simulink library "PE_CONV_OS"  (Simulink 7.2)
settings: Solver=ode45  SolverMode=SingleTasking  StartTime=0.0  StopTime=10.0  RelTol=1e-3
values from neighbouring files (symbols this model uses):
  C = 10e-3*1    (= 0.01)    [INIT_B6_2L_3Ph_IGBT_OS.m]    (also in INIT_B6_3L_3Ph_IGBT_OS.m; INIT_MMC_100L.m = 0.005; INIT_MMC_200L.m = 0.005; INIT_MMC_20L.m)
  FS = 900    [INIT_B6_2L_3Ph_IGBT_OS.m]    (also in INIT_B6_3L_3Ph_IGBT_OS.m; INIT_PWM_2L.m = 1000; INIT_PWM_3L.m = 1000; INIT_PWM_Con.m = 1000)
  LN = 2e-3    (= 0.002)    [INIT_PWM_2L.m]    (also in INIT_PWM_3L.m; INIT_PWM_Con.m; INIT_MMC_100L.m = 0.025; INIT_MMC_200L.m = 0.025)
  LS = 1e-3    (= 0.001)    [INIT_B6_2L_3Ph_IGBT_OS.m]    (also in INIT_B6_3L_3Ph_IGBT_OS.m; INIT_MMC_100L.m = 0.025; INIT_MMC_200L.m = 0.025; INIT_MMC_20L.m = 0.0025)
  LT = LN    (= 0.025)    [INIT_MMC_100L.m]    (also in INIT_MMC_200L.m; INIT_MMC_20L.m = 0.002; INIT_MMC_400L.m)
  Nc = 100    [INIT_MMC_100L.m]    (also in INIT_MMC_200L.m = 200; INIT_MMC_20L.m = 20; INIT_MMC_400L.m = 400)
  NT = sqrt(3)*340/400    [INIT_MMC_100L.m]    (also in INIT_MMC_200L.m; INIT_MMC_20L.m = sqrt(3); INIT_MMC_400L.m)
  Rg = 1e-3    (= 0.001)    [INIT_MMC_100L.m]    (also in INIT_MMC_200L.m; INIT_MMC_20L.m; INIT_MMC_400L.m)
  RN = 0.1    [INIT_PWM_2L.m]    (also in INIT_PWM_3L.m; INIT_PWM_Con.m; INIT_MMC_100L.m; INIT_MMC_200L.m)
  RT = RN    (= 0.1)    [INIT_MMC_100L.m]    (also in INIT_MMC_200L.m; INIT_MMC_20L.m; INIT_MMC_400L.m)
  UC0 = 600    [INIT_B6_2L_3Ph_IGBT_OS.m]    (also in INIT_B6_3L_3Ph_IGBT_OS.m = 500; INIT_MMC_100L.m = 6800; INIT_MMC_200L.m = 3400; INIT_MMC_20L.m = 5000)
undefined symbols (not defined in the file or in its folder): A, DT, FT, L, O1, O2, PHT, T, Td
libraries: simulink_extras x2
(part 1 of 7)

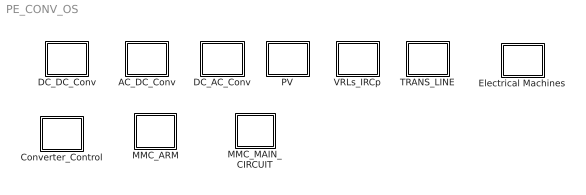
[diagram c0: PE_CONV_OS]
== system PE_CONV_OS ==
  AC_DC_Conv : Subsystem
  Converter_Control : Subsystem
  DC_AC_Conv : Subsystem
  DC_DC_Conv : Subsystem
  Electrical Machines : Subsystem
  MMC_ARM : Subsystem
  MMC_MAIN_CIRCUIT : Subsystem
  PV : Subsystem
  TRANS_LINE : Subsystem
  VRLs_IRCp : Subsystem

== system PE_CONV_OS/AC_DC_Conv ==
  B12D_OS : Subsystem  mask{LS=1e-4, nyy=1, nyd=sqrt(3), LT=1e-4, LD=1e-3, ILD0=200, C=1e-3, VC0=600, RL=2}
      mask prompts: LS "Source Inductance"; nyy "Trafo YY turns Ratio"; nyd "Trafo YD turns Ratio"; LT "Transformer Inductance"; LD "DC Inductance"; ILD0 "Initial Current ILD0"; C "Load Capacitance"; VC0 "Initial Cap Voltage"; RL "Load Resistance"
      mask help: 12-Pulse Diode Bridge Converter Input Vector u: u[0]= Vs1.v u[1]= Vs2.v u[2]= Vs3.v u[3]= IDC1.i u[4]= IDC2.i Output Vector y: y[0]= D11.I y[1]= D11.V y[2]= D12.I y[3]= D12.V y[4]= Lc1.I y[5]= Lc2.I y[6]= Lc3.I y[7]= Ld1.I y[8]= Ld2.I y[9]= VDC1.V y[10]= VDC2.V y[11]= VC1.V y[12]= VC2.V Parameter Vector p: p[0]= Lc1.L p[0]= Lc2.L p[0]= Lc3.L p[1]= nyy p[2]= nyd p[3]= LT.L p[4]= Ld.L p[5]= Ld.IL0 p[6]= C1.C p[7]= C1.vC0 p[8]= R1.r You can pause the simulation during running, change the Parameters you want and continue the Simulation
  B12T_OS : Subsystem  mask{LS=1e-4, LT1=1e-4, LT2=1e-4, LD=1e-3, ILD0=200, C=5e-3, VC0=500, RL=2}
      mask prompts: LS "source Inductance"; LT1 "TYY leakage Inductance"; LT2 "TYD leakage Inductance"; LD "DC Inductance"; ILD0 "Initial Current ILD0"; C "Load Capacitance"; VC0 "Initial Cap Voltage"; RL "Load Resistance"
      mask help: 12-Pulse Thyristor Bridge Converter Input Vector u: u[0]= B6T1_H1.gate u[1]= B6T1_H2.gate u[2]= B6T1_H3.gate u[3]= B6T1_H4.gate u[4]= B6T1_H5.gate u[5]= B6T1_H6.gate u[6]= B6T2_H1.gate u[7]= B6T2_H2.gate u[8]= B6T2_H3.gate u[9]= B6T2_H4.gate u[10]= B6T2_H5.gate u[11]= B6T2_H6.gate u[12]= Vs1.v u[13]= Vs2.v u[14]= Vs3.v u[15]= IDC1.i u[16]= IDC1.i Output Vector y: y[0]= B6T1_T11.I y[1]= B6T1_T11.V y[2]= B6T2_T11.I y[3]= B6T2_T11.V y[4]= Ls1.I y[5]= Ls2.I y[6]= Ls3.I y[7]= Ld1.I y[8]= Ld2.I y[6]= VDC.V y[9]= VC1.V y[10]= VC2.V Parameter Vector p: p[0]= Ls.L p[1]= TYY_LT.L p[2]= TYD_LT.L p[3]= Ld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
  B2D_OS : Subsystem  mask{LS=1e-3, LD=1e-3, ILD0=80, C=1e-5, VC0=80, RD=2}
      mask prompts: LS "Source Inductance"; LD "Load Inductance"; ILD0 "initial  Load Inductance Current"; C "Load Cap"; VC0 "initial Cap Voltage"; RD "Load Resistance"
      mask help: Open Source 2-Pulse Diode Bridge Converter Input Vector u: u[0]= Vs.v u[1]= IDC.i Output Vector y: y[0]= D1.I y[1]= D1.V y[2]= Lc.I y[3]= Ld.I y[4]= VDC.V y[5]= VC.V Parameter Vector p: p[0]= Lc.L p[1]= Ld.L p[2]= Ld.IL0 p[3]= C1.C p[4]= C1.vC0 p[5]= R1.r You can pause the simulation during running, change the Parameters you want and continue the Simulation
  B2T_OS : Subsystem  mask{LS=1e-4, LD=10e-3, ILD0=0, C=10e-3, VC0=100, RL=1}
      mask prompts: LS "Source Inductance"; LD "DC Inductance"; ILD0 "Initial current ILD0"; C "Load Cap"; VC0 "Initial Cap Voltage"; RL "Load Resistance"
      mask help: 2-Pulse Thyristor Bridge Converter Input Vector u: u[0]= H1.gate,H4.gate u[1]= H2.gate,H3.gate u[2]= Vs.v u[3]= IDC.i Output Vector y: y[0]= T1.I y[1]= T1.V y[2]= Lc.I y[3]= Ld.I y[4]= VDC.V y[5]= VC.V Parameter Vector p: p[0]= Lc.L p[1]= Ld.L p[2]= Ld.IL0 p[3]= C1.C p[4]= C1.vC0 p[5]= R1.r You can pause the simulation during running, change the Parameters you want and continue the Simulation
  B2_2L_IGBT_OS : Subsystem  mask(B2-2-Level IGBT Converter){LS=2e-3, C=10e-3, VC0=400, RL=10e5}
      mask prompts: LS "Source Inductance"; C "Load Cap"; VC0 "Initial Cap Voltage"; RL "Load Resistance"
      mask help: Input Vector u: u[0]= IGBT1.gate u[1]= IGBT2.gate u[2]= IGBT3.gate u[3]= IGBT4.gate u[4]= V1.V u[5]= IDC.i Output Vector y: y[0]= T1.I y[1]= D1.I y[2]= T1.V y[3]= T2.I y[4]= D2.I y[5]= T2.V y[6]= LS1.I y[7]= DC.V y[8]= Va.V Parameter Vector p: p[0]= Ls.L p[1]= C1.C p[2]= C1.vC0 p[3]= R1.r You can pause the simulation during running, change the Parameters you want and continue the Simulation
  B2_3LD_IGBT_OS : Subsystem  mask(B2-2-Level IGBT Converter){LS=2e-3, C=10e-3, VC0=200, RL=10e5}
      mask prompts: LS "Source Inductance"; C "Load Cap"; VC0 "Initial Cap Voltage"; RL "Load Resistance"
      mask help: Input Vector u: u[0]= IGBT1.gate u[1]= IGBT2.gate u[2]= IGBT3.gate u[3]= IGBT4.gate u[4]= V1.V u[5]= IDC.i Output Vector y: y[0]= T1.I y[1]= D1.I y[2]= T1.V y[3]= T2.I y[4]= D2.I y[5]= T2.V y[6]= LS1.I y[7]= DC.V y[8]= Va.V Parameter Vector p: p[0]= Ls.L p[1]= C1.C p[2]= C1.vC0 p[3]= R1.r You can pause the simulation during running, change the Parameters you want and continue the Simulation
  B2_3LT_IGBT_OS : Subsystem  mask(B2-2-Level IGBT Converter){LS=2e-3, C=10e-3, VC0=200, RL=10e5}
      mask prompts: LS "Source Inductance"; C "Load Cap"; VC0 "Initial Cap Voltage"; RL "Load Resistance"
      mask help: Input Vector u: u[0]= IGBT1.gate u[1]= IGBT2.gate u[2]= IGBT3.gate u[3]= IGBT4.gate u[4]= V1.V u[5]= IDC.i Output Vector y: y[0]= T1.I y[1]= D1.I y[2]= T1.V y[3]= T2.I y[4]= D2.I y[5]= T2.V y[6]= LS1.I y[7]= DC.V y[8]= Va.V Parameter Vector p: p[0]= Ls.L p[1]= C1.C p[2]= C1.vC0 p[3]= R1.r You can pause the simulation during running, change the Parameters you want and continue the Simulation
  B6D_OS : Subsystem  mask{LS=1e-4, LD=1e-3, ILD0=200, C=1e-3, VC0=500, RL=2}
      mask prompts: LS "Source Inductance"; LD "DC Inductance"; ILD0 "Initial current ILD0"; C "Load Cap"; VC0 "Initial Cap Voltage"; RL "Load Resistance"
      mask help: 6-Pulse Diode Bridge Converter Input Vector u: u[0]= Vs1.v u[1]= Vs2.v u[2]= Vs3.v u[3]= IDC.i Output Vector y: y[0]= D1.I y[1]= D1.V y[2]= Lc1.I y[3]= Lc2.I y[4]= Lc3.I y[5]= Ld.I y[6]= VDC.V y[7]= VC.V Parameter Vector p: p[0]= Lc1.L p[0]= Lc2.L p[0]= Lc3.L p[1]= Ld.L p[2]= Ld.IL0 p[3]= C1.C p[4]= C1.vC0 p[5]= R1.r You can pause the simulation during running, change the Parameters you want and continue the Simulation
  B6T_OS : Subsystem  mask{LS=1e-4, LD=1e-3, ILD0=200, C=2e-3, VC0=500, RL=2}
      mask prompts: LS "Source Inductance"; LD "DC Inductance LD"; ILD0 "Initial current ILD0"; C "Load Cap"; VC0 "Initial Cap Voltage"; RL "Load Resistance"
      mask help: 6-Pulse Thyristor Bridge Converter Input Vector u: u[0]= H1.gate u[1]= H2.gate u[2]= H3.gate u[3]= H4.gate u[4]= H5.gate u[5]= H6.gate u[6]= Vs1.v u[7]= Vs2.v u[8]= Vs3.v u[9]= IDC.i Output Vector y: y[0]= T11.I y[1]= T11.V y[2]= Lc1.I y[3]= Lc2.I y[4]= Lc3.I y[5]= Ld.I y[6]= VDC.V y[7]= VC.V Parameter Vector p: p[0]= Lc.L p[1]= Ld.L p[2]= Ld.IL0 p[3]= C1.C p[4]= C1.vC0 p[5]= R1.r You can pause the simulation during running, change the Parameters you want and continue the Simulation
  B6_2L_3ph_IS_IGBT_OS : Subsystem  mask(B6 2-Level IGBT 3-Phase Converter){C=C, UC0=UC0, RL=10000}
      mask prompts: C "Load Cap"; UC0 "Initial Cap Voltage"; RL "Load Resistance"
      mask help: Input Vector u: u[0]= IGBT1.gate u[1]= IGBT2.gate u[2]= IGBT3.gate u[3]= IGBT4.gate u[4]= IGBT5.gate u[5]= IGBT6.gate u[6]= I1.V u[7]= I2.V u[8]= I3.V u[9]= IDC Output Vector y: y[0]= T1.I y[1]= D1.I y[2]= T1.V y[3]= T2.I y[4]= D2.I y[5]= T2.V y[6]= DC.V y[7]= Va.V y[9]= Vb.V y[10]= Vc.V Parameter Vector p: p[0]= C1.C p[1]= C1.vC0 p[2]= R1.r You can pause the simulation during running, change the Parameters you want and continue the Simulation
  B6_2L_3ph_VLS_IGBT_OS : Subsystem  mask(B6 2-Level IGBT 3-Phase Converter){LS=LS, C=C, UC0=UC0, RL=10000}
      mask prompts: LS "Source Inductance"; C "Load Cap"; UC0 "Initial Cap Voltage"; RL "Load Resistance"
      mask help: Input Vector u: u[0]= IGBT1.gate u[1]= IGBT2.gate u[2]= IGBT3.gate u[3]= IGBT4.gate u[4]= IGBT5.gate u[5]= IGBT6.gate u[6]= V1.V u[7]= V2.V u[8]= V3.V u[9]= IDC.i Output Vector y: y[0]= T1.I y[1]= D1.I y[2]= T1.V y[3]= T2.I y[4]= D2.I y[5]= T2.V y[6]= LS1.I y[7]= LS2.I y[8]= LS3.I y[9]= DC.V y[10]= Va.V y[11]= Vb.V y[12]= Vc.V Parameter Vector p: p[0]= Ls.L p[1]= C1.C p[2]= C1.vC0 p[3]= R1.r You can pause the simulation during running, change the Parameters you want and continue the Simulation
  B6_3LD_3-ph_IGBT_OS : Subsystem  mask(6-Pulse 3-LD IGBT 3-Phase Converter){LS=LS, C=C, VC0=UC0, RL=1000}
      mask prompts: LS "Source Inductance"; C "Load Cap"; VC0 "Initial Cap Voltage"; RL "Load Resistance"
      mask help: Input Vector u: u[0]= IGBT1.gate u[1]= IGBT2.gate u[2]= IGBT3.gate u[3]= IGBT4.gate u[4]= IGBT5.gate u[5]= IGBT6.gate u[6]= IGBT7.gate u[7]= IGBT8.gate u[8]= IGBT9.gate u[9]= IGBT10.gate u[10]= IGBT11.gate u[11]= IGBT12.gate u[12]= V1.V u[13]= V2.V u[14]= V3.V u[15]= IDC.i Output Vector y: y[0]= T1.I y[1]= D1.I y[2]= T1.V y[3]= T2.I y[4]= D2.I y[5]= T2.V y[6]= LS1.I y[7]= LS2.I y[8]= LS3.I y[9]= DC1.V y[10]= DC2.V y[11]= Vab.V Parameter Vector p: p[0]= Ls.L p[1]= C1.C p[2]= C1.vC0 p[3]= R1.r You can pause the simulation during running, change the Parameters you want and continue the Simulation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
  B6_3LT_3-ph_IGBT_OS : Subsystem  mask(6-Pulse 3-LT IGBT 3-Phase Converter){LS=LS, C=C, VC0=UC0, RL=1000}
      mask prompts: LS "Source Inductance"; C "Load Cap"; VC0 "Initial Cap Voltage"; RL "Load Resistance"
      mask help: Input Vector u: u[0]= IGBT1.gate u[1]= IGBT2.gate u[2]= IGBT3.gate u[3]= IGBT4.gate u[4]= IGBT5.gate u[5]= IGBT6.gate u[6]= IGBT7.gate u[7]= IGBT8.gate u[8]= IGBT9.gate u[9]= IGBT10.gate u[10]= IGBT11.gate u[11]= IGBT12.gate u[12]= V1.V u[13]= V2.V u[14]= V3.V u[15]= IDC.i Output Vector y: y[0]= T1.I y[1]= D1.I y[2]= T1.V y[3]= T2.I y[4]= D2.I y[5]= T2.V y[6]= LS1.I y[7]= LS2.I y[8]= LS3.I y[9]= DC1.V y[10]= DC2.V y[11]= Vab.V Parameter Vector p: p[0]= Ls.L p[1]= C1.C p[2]= C1.vC0 p[3]= R1.r You can pause the simulation during running, change the Parameters you want and continue the Simulation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

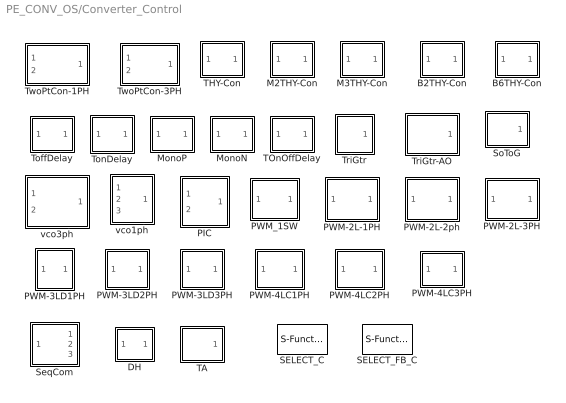
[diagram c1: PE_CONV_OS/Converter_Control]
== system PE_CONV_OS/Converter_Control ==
  B2THY-Con : Subsystem  mask(B2THY-Con){F=50, PH=90, TD=1e-3}
      mask prompts: F "Frequency"; PH "Phase Angle (Degree)"; TD "Puls Duration"
      mask help: Control of one Thyristor in a line commutated Converter circuit
      mask init:
      | x=0:pi/20:2*pi;
      | y=cos(x);
  B6THY-Con : Subsystem  mask(B6THY-Con){F=50, PH=60, TD=1e-3}
      mask prompts: F "Frequency"; PH "Phase Angle (Degree)"; TD "Puls Duration"
      mask help: Control of one Thyristor in a line commutated Converter circuit
      mask init:
      | x=0:pi/20:2*pi;
      | y=cos(x);
  DH : Subsystem
  M2THY-Con : Subsystem  mask(M1THY-Con){F=50, PH=90, TD=1e-3}
      mask prompts: F "Frequency"; PH "Phase Angle (Degree)"; TD "Puls Duration"
      mask help: Control of one Thyristor in a line commutated Converter circuit
      mask init:
      | x=0:pi/20:2*pi;
      | y=cos(x);
  M3THY-Con : Subsystem  mask(M3THY-Con){F=50, PH=60, TD=1e-3}
      mask prompts: F "Frequency"; PH "Phase Angle (Degree)"; TD "Puls Duration"
      mask help: Control of one Thyristor in a line commutated Converter circuit
      mask init:
      | x=0:pi/20:2*pi;
      | y=cos(x);
  MonoN : Subsystem  mask(MonoN){PW=1e-6}
      mask prompts: PW "Pulse Width"
      mask help: Mono Flip Flop on nagative going signal
  MonoP : Subsystem  mask(MonoP){PW=1e-6}
      mask prompts: PW "Pulse Width"
      mask help: Mono Flip Flop on positive going signal
  PIC : Subsystem  mask(PI-controller){Kp=1, Ki=10, lim=15, Ts=-1}
      mask prompts: Kp "Proportional gain (Kp)"; Ki "Integral gain (Ki)"; lim "Output limit"; Ts "Sampling time (s)"
      mask help: Proportional-Integral Controller
  PWM-2L-1PH : Subsystem  mask(PWM-2L-1PH){FT=5000, PHT=0, DT=1e-6}
      mask prompts: FT "Triangular Frequency"; PHT "Trian. Phase Angle (Degree)"; DT "Dead Time"
      mask help: Pulse Width Modulation for 1 Leg of 2-Level Converter
  PWM-2L-2ph : Subsystem  mask(PWM-2L-2PH){FT=500, PHT=0, DT=1e-6}
      mask prompts: FT "Triangular Frequency"; PHT "Trian. Phase Angle (Degree)"; DT "Dead Time"
      mask help: Pulse Width Modulation for 2 Legs of 2-Level Converter
  PWM-2L-3PH : Subsystem  mask(PWM3-2L-3PH){FT=500, PHT=0, DT=1e-6}
      mask prompts: FT "Triangular Frequency"; PHT "Trian. Phase Angle (Degree)"; DT "Dead Time"
      mask help: Pulse Width Modulation for 3 Phase Converter
  PWM-3LD1PH : Subsystem  mask(PWM-3LD_1PH){FT=FT, PHT=PHT, A=A, O1=O1, O2=O2, DT=DT}
      mask prompts: FT "Frequency of Trian Sig."; PHT "Phase Angle of Trian. Sig."; A "Amplitude of Trian. Sig."; O1 "Offset of 1st Trian"; O2 "Offset of 2nd Trian."; DT "Dead Time"
      mask help: Pulse Width Modulation for 1 Leg of 3 Level Neutral point clamped Converter
  PWM-3LD2PH : Subsystem  mask(PWM-3LD_3PH){FT=5000, PHT=0, A=0.5, O1=0.5, O2=-0.5, DT=1e-6}
      mask prompts: FT "Frequency of Trian Sig."; PHT "Phase Angle of Trian. Sig."; A "Amplitude of Trian. Sig."; O1 "Offset of 1st Trian"; O2 "Offset of 2nd Trian."; DT "Dead Time"
      mask help: Pulse Width Modulation for 2 Legs of 3 Level Neutral point clamped Converter
  PWM-3LD3PH : Subsystem  mask(PWM-3LD3PH){FT=500, PHT=0, A=0.5, O1=0.5, O2=-0.5, DT=1e-6}
      mask prompts: FT "Frequency of Trian Sig."; PHT "Phase Angle of Trian. Sig."; A "Amplitude of Trian. Sig."; O1 "Offset of 1st Trian"; O2 "Offset of 2nd Trian."; DT "Dead Time"
      mask help: Pulse Width Modulation for 3 Phase 3 Level Neutral point clamped Converter
  PWM-4LC1PH : Subsystem  mask(PWM-4LC1PH){FT=500, PHT1=0, PHT2=-120, PHT3=-240, DT=1e-6}
      mask prompts: FT "Frequency of Trian Sig."; PHT1 "Phase Angle of 1st Trian. Sig."; PHT2 "Phase Angle of 2nd Trian. Sig."; PHT3 "Phase Angle of 3rd Trian. Sig."; DT "Dead Time"
      mask help: Pulse Width Modulation for 1 Phase 4 Level Floating Capacitor Converter
  PWM-4LC2PH : Subsystem  mask(PWM-4LC1PH){FT=500, PHT1=0, PHT2=-120, PHT3=-240, DT=1e-6}
      mask prompts: FT "Frequency of Trian Sig."; PHT1 "Phase Angle of 1st Trian. Sig."; PHT2 "Phase Angle of 2nd Trian. Sig."; PHT3 "Phase Angle of 3rd Trian. Sig."; DT "Dead Time"
      mask help: Pulse Width Modulation for 1 Phase 4 Level Floating Capacitor Converter
  PWM-4LC3PH : Subsystem  mask(PWM-4LC3PH){FT=500, PHT1=0, PHT2=-120, PHT3=-240, DT=1e-6}
      mask prompts: FT "Frequency of Trian Sig."; PHT1 "Phase Angle of 1st Trian. Sig."; PHT2 "Phase Angle of 2nd Trian. Sig."; PHT3 "Phase Angle of 3rd Trian. Sig."; DT "Dead Time"
      mask help: Pulse Width Modulation for 3 Phases 4 Level Floating Capacitor Converter
  PWM_1SW : Subsystem  mask(PWMtr){FS=1000}
      mask prompts: FS "Frequency"
      mask help: PWM based on Saw tooth Generator
  SELECT_C : S-Function  FunctionName=SELECT_MMC_C  Parameters=2*Nc  EnableBusSupport=off
  SELECT_FB_C : S-Function  FunctionName=SELECT_MMC_AFB_C  Parameters=2*Nc  EnableBusSupport=off
  SeqCom : Subsystem  mask{T=0.02, BF=1024*10}
      mask prompts: T "Period Time"; BF "Beffer Size"
      mask help: Unbalaced 3-phase system to Positive, Negative and Zero Sequence Systems
  SoToG : Subsystem  mask(SoToG){T=1e-3}
      mask prompts: T "Period Time"
      mask help: Saw tooth Generator Input: Period Time
  TA : Subsystem  mask(TriGtr-AO){A=0.5, O=0.5, T=1/FS, Nc=Nc}
      mask prompts: A "Amplitude"; O "Offset"; T "Period Time"; Nc "Output width"
      mask help: Triangular Wave Generator with variable No. of triagles, variable amplitude and offset
  THY-Con : Subsystem  mask(THY-Con){F=50, PH=90, TD=1e-3}
      mask prompts: F "Frequency"; PH "Phase Angle (Degree)"; TD "Puls Duration"
      mask init:
      | x=0:pi/20:2*pi;
      | y=cos(x);
  TOnOffDelay : Subsystem  mask(TOnOffDelay){DT_OFF=1e-6, DT_ON=1e-6}
      mask prompts: DT_OFF "TOffDelay"; DT_ON "TOnDelay"
  ToffDelay : Subsystem  mask(TOffDelay){DT=1e-6}
      mask prompts: DT "TOffDelay"
  TonDelay : Subsystem  mask(TonDelay){DT=1e-6}
      mask prompts: DT "Dead Time"
      mask help: Turn on dead time to protect against short circuit of the converter leg
  TriGtr : Subsystem  mask(TriGtr){T=1e-3, Td=0.0002}
      mask prompts: T "Period Time"; Td "Time Delay"
      mask help: Triangular Wave Generator with variable time delay
  TriGtr-AO : Subsystem  mask(TriGtr-AO){A=0.5, O=0.5, T=T, Td=Td}
      mask prompts: A "Amplitude"; O "Offset"; T "Period Time"; Td "Time Delay"
      mask help: Triangular Wave Generator with variable time delay, variable amplitude and offset
  TwoPtCon-1PH : Subsystem  mask(TwoPtCon-1PH){SP=5, SN=-5, DT=1e-6}
      mask prompts: SP "Positive Limit"; SN "Negative Limit"; DT "Dead Time"
      mask help: Two Point Controller with Dead Time protection for 1Phase Converter
  TwoPtCon-3PH : Subsystem  mask(TwoPtCon-3PH){SP=5, SN=-5, DT=1e-6}
      mask prompts: SP "Positive Limit"; SN "Negative Limit"; DT "Dead Time"
      mask help: Two Point Controller with Dead Time protection for 3 Phase Converter
  vco1ph : Subsystem
  vco3ph : Subsystem

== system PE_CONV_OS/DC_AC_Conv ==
  PWM_2L_3PH_IS : Subsystem
  PWM_2L_3PH_VLR : Subsystem  mask(pwm_2L_3PH_VLR_OS){RL=0.5, LL=1e-3}
      mask prompts: RL "Load R"; LL "Load L"
      mask help: Open Source 2-Level PWM_3PH Converter with VLR load Input Vector u: u[0]= TD1.gate u[1]= TD2.gate u[2]= TD3.gate u[3]= TD4.gate u[4]= TD5.gate u[5]= TD6.gate u[6]= VDC u[7]= Ea, Phase A Load Voltage u[8]= Eb, Phase B Load Voltage u[9]= Ec, Phase C Load Voltage Output Vector y: y[0]= Va.v, Phase A Output Voltage to middle point y[1]= Vb.V, Phase B Output Voltage to middle point y[2]= Vc.V, Phase C Output Voltage to middle point y[3]= Ia.I, Phase A Output AC Current y[4]= Ib.I, Phase B Output AC Current y[5]= Ic.I, Phase C Output AC Current y[6]= Vab.V, Output AC line Voltage y[7]= T1.I y[8]= D1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
  PWM_2L_FB_IS : Subsystem
  PWM_2L_FB_VLR : Subsystem  mask(pwm_2L_FB_VLR_OS){RL=1, LL=1e-3}
      mask prompts: RL "Load R"; LL "Load L"
      mask help: Open Source 2-Level FB_PWM Converter with VLR load Input Vector u: u[0]= TD1.gate u[1]= TD2.gate u[2]= TD3.gate u[3]= TD4.gate u[4]= VDC u[5]= EL, Load Voltage Output Vector y: y[0]= Va.v, Output Voltage to middle point y[1]= Ia.I, Output AC Current y[2]= Vab.V, Output AC Voltage y[3]= T1.I y[4]= D1.I y[5]= T1.V y[6]= DC.I, Input DC Current Parameter Vector p: p[0]= RL p[1]= LL You can pause the simulation during running, change the Parameters you want and continue the Simulation
  PWM_2L_HB_IS : Subsystem
  PWM_2L_HB_VLR : Subsystem  mask(pwm_2L_HB_VLR_OS){RL=0.5, LL=1e-3}
      mask prompts: RL "Load R"; LL "Load L"
      mask help: Open Source 2-Level HB_PWM Converter with VLR load Input Vector u: u[0]= TD1.gate u[1]= TD2.gate u[2]= VDC u[3]= Ea Output Vector y: y[0]= Va.v, Output Voltage to middle point y[1]= Ia.I, Output AC Current y[2]= T1.I y[3]= D1.I y[4]= T1.V y[5]= DC.I, Input DC Current Parameter Vector p: p[0]=RL p[1]=LL You can pause the simulation during running, change the Parameters you want and continue the Simulation
  PWM_3LD_3PH_IS : Subsystem
  PWM_3LD_3PH_VLR : Subsystem  mask(pwm_3LD_3PH_VLR_OS){RL=1, LL=1e-3}
      mask prompts: RL "Load Resistance"; LL "Load Inductance"
      mask help: Open Source 3-Level NPC PWM_3PH Converter with VLR load Input Vector u: u{0:11}= gating Signals u[12]/2= VDC1, VDC2 u{13:15}= EA,EB,EC Output Vector y: y{0:2}= Va,Vb,Vc, Output AC Voltages to middle point y{3:5}= Ia,Ib,Ic, Output AC Currents y[6]= Vab.V, Output Voltage y{7:9} = T1.I,D1.I,T1.V y{10:12}= T2.I,D2.I,T2.V y[13]= D5.I y[14]= D5.V y[15]= IDC1, Input DC Current y[16]= IDC2, Input DC Current Parameter Vector p: p[0]=RL p[1]=LL You can pause the simulation during running, change the Parameters you want and continue the Simulation
  PWM_3LD_FB_IS : Subsystem
  PWM_3LD_FB_VLR : Subsystem  mask(pwm_3LD_FB_VLR_OS){RL=1, LL=1e-3}
      mask prompts: RL "Load Resistance"; LL "Load Inductance"
      mask help: Open Source 3-Level NPC Full Bridge Converter with VLR load Input Vector u: u[0]= L3L1_TD1.gate u[1]= L3L1_TD2.gate u[2]= L3L1_TD3.gate u[3]= L3L1_TD4.gate u[4]= L3L2_TD1.gate u[5]= L3L2_TD2.gate u[6]= L3L2_TD3.gate u[7]= L3L2_TD4.gate u[8]= VDC u[9]= EL Output Vector y: y[0]= Va.v, Output AC Voltage to middle point y[1]= Ia.I, Output AC Current y[2]= Vab.V, Output AC Voltage y[3]= T1.I y[4]= D1.I y[5]= T1.V y[6]= T2.I y[7]= D2.I y[8]= T2.V y[9]= D5.I y[10]= D5.V y[11]= IDC1, Input DC Current y[12]= IDC2, Input DC Current Parameter Vector p: p[0]=RL p[1]=LL You can pause the simulation during 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
  PWM_3LD_HB_IS : Subsystem
  PWM_3LD_HB_VLR : Subsystem  mask(pwm_3LD_HB_VLR_OS){RL=0.5, LL=2e-3}
      mask prompts: RL "Load Resistance"; LL "Load Inductance"
      mask help: Open Source 3-Level NPC PWM HB Converter with VLR load Input Vector u: u[0]= L3L1_TD1.gate u[1]= L3L1_TD2.gate u[2]= L3L1_TD3.gate u[3]= L3L1_TD4.gate u[4]= VDC u[5]= Ea Output Vector y: y[0]= Va.v, Output Voltage to middle point y[1]= Ia.I, Output AC Current y[2]= T1.I y[3]= D1.I y[4]= T1.V y[5]= T2.I y[6]= D2.I y[7]= T2.V y[8]= D5.I y[9]= D5.V y[10]= IDC1, Input DC Current y[11]= IDC2, Input DC Current Parameter Vector p: p[0]=RL p[1]=LL You can pause the simulation during running, change the Parameters you want and continue the Simulation
  PWM_3LT_3PH_IS : Subsystem
  PWM_3LT_3PH_VLR : Subsystem  mask(pwm_3LT_3PH_VLR_OS){RL=1, LL=1e-3}
      mask prompts: RL "Load Resistance"; LL "Load Inductance"
      mask help: Open Source 3-Level T-NPC PWM_3PH Converter with VLR load Input Vector u: u{0:11}= gating Signals u[12]/2= VDC1, VDC2 u{13:15}= EA,EB,EC Output Vector y: y{0:2}= Va,Vb,Vc, Output AC Voltages to middle point y{3:5}= Ia,Ib,Ic, Output AC Currents y[6]= Vab.V, Output Voltage y{7:9} = T1.I,D1.I,T1.V y{10:12}= T2.I,D2.I,T2.V y[13]= D5.I y[14]= D5.V y[15]= IDC1, Input DC Current y[16]= IDC2, Input DC Current Parameter Vector p: p[0]=RL p[1]=LL You can pause the simulation during running, change the Parameters you want and continue the Simulation
  PWM_3LT_FB_IS : Subsystem
  PWM_3LT_FB_VLR : Subsystem  mask(pwm_3LT_FB_VLR_OS){RL=1, LL=1e-3}
      mask prompts: RL "Load Resistance"; LL "Load Inductance"
      mask help: Open Source 3-Level T-NPC Full Bridge Converter Input Vector u: u[0]= L3L1_TD1.gate u[1]= L3L1_TD2.gate u[2]= L3L1_TD3.gate u[3]= L3L1_TD4.gate u[4]= L3L2_TD1.gate u[5]= L3L2_TD2.gate u[6]= L3L2_TD3.gate u[7]= L3L2_TD4.gate u[8]= VDC u[9]= EL Output Vector y: y[0]= Va.v, Output AC Voltage to middle point y[1]= Ia.I, Output AC Current y[2]= Vab.V, Output AC Voltage y[3]= T1.I y[4]= D1.I y[5]= T1.V y[6]= T2.I y[7]= D2.I y[8]= T2.V y[9]= D5.I y[10]= D5.V y[11]= IDC1, Input DC Current y[12]= IDC2, Input DC Current Parameter Vector p: p[0]=RL p[1]=LL You can pause the simulation during running, cha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
  PWM_3LT_HB_IS : Subsystem
  PWM_3LT_HB_VLR : Subsystem  mask(pwm_3LD_HB_VLR_OS){RL=1, LL=1e-3}
      mask prompts: RL "Load Resistance"; LL "Load Inductance"
      mask help: Open Source 3-Level T-NPC PWM HB Converter with VLR load Input Vector u: u[0]= L3L1_TD1.gate u[1]= L3L1_TD2.gate u[2]= L3L1_TD3.gate u[3]= L3L1_TD4.gate u[4]= VDC u[5]= EA Output Vector y: y[0]= Va.v, Output Voltage to middle point y[1]= Ia.I, Output AC Current y[2]= T1.I y[3]= D1.I y[4]= T1.V y[5]= T2.I y[6]= D2.I y[7]= T2.V y[8]= D5.I y[9]= D5.V y[10]= IDC1, Input DC Current y[11]= IDC2, Input DC Current Parameter Vector p: p[0]=RL p[1]=LL You can pause the simulation during running, change the Parameters you want and continue the Simulation
  PWM_4LC_3PH_IS : Subsystem  mask(pwm_4LC_3PH_IS_OS){C1=10e-3, VC10=2*1500/3, C2=10e-3, VC20=1500/3}
      mask prompts: C1 "Cap C1"; VC10 "Initial Cap Voltage VC10"; C2 "Cap C2"; VC20 "Initial Cap Voltage VC20"
      mask help: Open Source 4-Level FC PWM 3PH Converter with IS load Input Vector u: u[0]= L4LC1_TD1.gate u[1]= L4LC1_TD2.gate u[2]= L4LC1_TD3.gate u[3]= L4LC1_TD4.gate u[4]= L4LC1_TD5.gate u[5]= L4LC1_TD6.gate u[6]= L4LC2_TD1.gate u[7]= L4LC2_TD2.gate u[8]= L4LC2_TD3.gate u[9]= L4LC2_TD4.gate u[10]= L4LC2_TD5.gate u[11]= L4LC2_TD6.gate u[12]= L4LC3_TD1.gate u[13]= L4LC3_TD2.gate u[14]= L4LC3_TD3.gate u[15]= L4LC3_TD4.gate u[15]= L4LC3_TD5.gate u[17]= L4LC3_TD6.gate u[18]= VDC u[19]= IA, Phase A Load Current as AC Current source u[20]= IB, Phase B Load Current as AC Current source Output Vector y: y[0]= Va.v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
  PWM_4LC_3PH_VLR : Subsystem  mask(pwm_4LC_3PH_VLR_OS){C1=10e-3, VC10=2*1500/3, C2=10e-3, VC20=1500/3, RL=1, LL=1e-3}
      mask prompts: C1 "Cap C1"; VC10 "Initial Cap Voltage VC10"; C2 "Cap C2"; VC20 "Initial Cap Voltage VC20"; RL "Load Res."; LL "Load Ind."
      mask help: Open Source 4-Level FC PWM 3PH Converter with VLR load Input Vector u: u[0]= L4LC1_TD1.gate u[1]= L4LC1_TD2.gate u[2]= L4LC1_TD3.gate u[3]= L4LC1_TD4.gate u[4]= L4LC1_TD5.gate u[5]= L4LC1_TD6.gate u[6]= L4LC2_TD1.gate u[7]= L4LC2_TD2.gate u[8]= L4LC2_TD3.gate u[9]= L4LC2_TD4.gate u[10]= L4LC2_TD5.gate u[11]= L4LC2_TD6.gate u[12]= L4LC3_TD1.gate u[13]= L4LC3_TD2.gate u[14]= L4LC3_TD3.gate u[15]= L4LC3_TD4.gate u[15]= L4LC3_TD5.gate u[17]= L4LC3_TD6.gate u[18]= VDC u[19]= EA u[20]= EB u[21]= EC Output Vector y: y[0]= Va.v, Phase A Output AC Voltage to middle point y[1]= Vb.V, Phase B Output AC V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
  PWM_4LC_FB_IS : Subsystem  mask(pwm_4LC_FB_IS_OS){C1=10e-3, VC10=2*1500/3, C2=10e-3, VC20=1500/3}
      mask prompts: C1 "Cap C1"; VC10 "Initial Cap Voltage VC10"; C2 "Cap C2"; VC20 "Initial Cap Voltage VC20"
      mask help: Open Source 4-Level FC PWM FB Converter with IS load Input Vector u: u[0]= TD1.gate u[1]= TD2.gate u[2]= TD3.gate u[3]= TD4.gate u[4]= TD5.gate u[5]= TD6.gate u[6]= TD7.gate u[7]= TD8.gate u[8]= TD9.gate u[9]= TD10.gate u[10]= TD11.gate u[11]= TD12.gate u[12]= VDC u[13]= IA, Load Current as AC Current source Output Vector y: y[0]= Va.v, Output AC Voltage to middle point y[1]= Ia.I, Output AC Current y[2]= T1.I y[3]= D1.I y[4]= T1.V y[5]= T2.I y[6]= D2.I y[7]= T2.V y[8]= T3.I y[9]= D3.I y[10]= T3.V y[11]= IDC1, Input DC Current y[12]= IDC2, Input DC Current Parameter Vector p: p[0]= C1 p[1]= VC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
  PWM_4LC_FB_VLR : Subsystem  mask(pwm_4LC_FB_VLR_OS){C1=10e-3, VC10=2*1500/3, C2=10e-3, VC20=1500/3, R1=5, L1=1e-3}
      mask prompts: C1 "Cap C1"; VC10 "Initial Cap Voltage VC10"; C2 "Cap C2"; VC20 "Initial Cap Voltage VC20"; R1 "Load Res"; L1 "Load Ind"
      mask help: Open Source 4-Level FC PWM FB Converter with IS load Input Vector u: u[0]= TD1.gate u[1]= TD2.gate u[2]= TD3.gate u[3]= TD4.gate u[4]= TD5.gate u[5]= TD6.gate u[6]= TD7.gate u[7]= TD8.gate u[8]= TD9.gate u[9]= TD10.gate u[10]= TD11.gate u[11]= TD12.gate u[12]= VDC u[13]= IA, Load Current as AC Current source Output Vector y: y[0]= Va.v, Output AC Voltage to middle point y[1]= Ia.I, Output AC Current y[2]= T1.I y[3]= D1.I y[4]= T1.V y[5]= T2.I y[6]= D2.I y[7]= T2.V y[8]= T3.I y[9]= D3.I y[10]= T3.V y[11]= IDC1, Input DC Current y[12]= IDC2, Input DC Current Parameter Vector p: p[0]= C1 p[1]= VC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
  PWM_4LC_HB_IS : Subsystem  mask(pwm_4LC_FB_IS_OS){C1=10e-3, VC10=2*1500/3, C2=10e-3, VC20=1500/3}
      mask prompts: C1 "Cap C1"; VC10 "Initial Cap Voltage VC10"; C2 "Cap C2"; VC20 "Initial Cap Voltage VC20"
      mask help: Open Source 4-Level FC PWM FB Converter with IS load Input Vector u: u[0]= TD1.gate u[1]= TD2.gate u[2]= TD3.gate u[3]= TD4.gate u[4]= TD5.gate u[5]= TD6.gate u[7]= VDC u[8]= IA, Load Current as AC Current source Output Vector y: y[0]= Va.v, Output AC Voltage to middle point y[1]= Ia.I, Output AC Current y[2]= T1.I y[3]= D1.I y[4]= T1.V y[5]= T2.I y[6]= D2.I y[7]= T2.V y[8]= T3.I y[9]= D3.I y[10]= T3.V y[11]= IDC1, Input DC Current y[12]= IDC2, Input DC Current Parameter Vector p: p[0]= C1 p[1]= VC10 p[2]= C2 p[3]= VC20 You can pause the simulation during running, change the Parameters you wan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
  PWM_4LC_HB_VLR : Subsystem  mask(pwm_4LC_3PH_VLR_OS){C1=10e-3, VC10=2*1500/3, C2=10e-3, VC20=1500/3, R1=2, L1=1e-3}
      mask prompts: C1 "Cap C1"; VC10 "Initial Cap Voltage VC10"; C2 "Cap C2"; VC20 "Initial Cap Voltage VC20"; R1 "Load Res."; L1 "Load Ind."
      mask help: Open Source 4-Level FC PWM HB Converter with VLR load Input Vector u: u[0]= L4LC1_TD1.gate u[1]= L4LC1_TD2.gate u[2]= L4LC1_TD3.gate u[3]= L4LC1_TD4.gate u[4]= L4LC1_TD5.gate u[5]= L4LC1_TD6.gate u[6]= VDC u[7]= VL Load Voltage as AC Voltage source Output Vector y: y[0]= Va.v Output AC Voltage to middle point y[1]= Ia.I Output AC Current y[2]= T1.I y[3]= D1.I y[4]= T1.V y[5]= T2.I y[6]= D2.I y[7]= T2.V y[8]= T3.I y[9]= D3.I y[10]= T3.V y[11]= IDC1, Input DC Current y[12]= IDC2, Input DC Current Parameter Vector p: p[0]= C1 p[1]= VC10 p[2]= C2 p[3]= VC20 p[4]= R1 p[5]= L1 You can pause the simu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

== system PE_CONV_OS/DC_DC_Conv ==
  BOOST_OS : Subsystem  mask{L1=10e-3, IL0=40, C1=1e-3, UC0=1200, R1=1e5}
      mask prompts: L1 "Inductance L1"; IL0 "Initial Current"; C1 "Capacitance"; UC0 "Initial Voltage"; R1 "Load Resistance"
      mask help: Open Source boost Converter Input Vector u: u[0]= T1.gate u[1]= E.v u[2]= IDC.i Output Vector y: y[0]= T1.I y[1]= D1.I y[2]= L1.I y[3]= C1.V Parameter Vector p: p[0]= L1.L p[1]= L1.iL0 p[2]= C1.C p[3]= C1.vC0 p[4]= R1.r You can pause the simulation during running, change the Parameters you want and continue the Simulation
  BUCK_BOOST_OS : Subsystem  mask{L1=10e-3, IL0=25, C1=5e-4, UC0=-105, R1=5}
      mask prompts: L1 "Inductance L1"; IL0 "Initial Current"; C1 "Capacitance"; UC0 "Initial Voltage"; R1 "Load Resistance"
      mask help: Open source Buck_boost Converter Input Vector u: u[0]= T1.gate u[1]= E.v u[2]= IDC.i Output Vector y: y[0]= T1.I y[1]= D1.I y[2]= L1.I y[3]= C1.V Parameter Vector p: p[0]= L1.L p[1]= L1.iL0 p[2]= C1.C p[3]= C1.vC0 p[4]= R1.r You can pause the simulation during running, change the Parameters you want and continue the Simulation
  BUCK_OS : Subsystem  mask{L1=5e-3, IL0=50, C1=5e-4, UC0=50, R1=1}
      mask prompts: L1 "Inductance L1"; IL0 "Initial Current"; C1 "Capacitance"; UC0 "Initial Voltage"; R1 "Load Resistance"
      mask help: Open source Buck Converter Input Vector u: u[0]= T1.gate u[1]= E.v u[2]= IDC.i Output Vector y: y[0]= T1.I y[1]= D1.I y[2]= L1.I y[3]= C1.V Parameter Vector p: p[0]= L1.L p[1]= L1.iL0 p[2]= C1.C p[3]= C1.vC0 p[4]= R1.r You can pause the simulation during running, change the Parameters you want and continue the Simulation
  FB4Q_OS : Subsystem  mask{L=5e-3, IL0=30, C=2e-4, VC0=50, R=10}
      mask prompts: L "Inductance L"; IL0 "Initial Current"; C "Cap"; VC0 "Initial Cap Voltage"; R "Load Resistance"
      mask help: Full Bridge 4Q Converter Input Vector u: u[0]= T1.gate u[1]= T2.gate u[2]= T3.gate u[3]= T4.gate u[4]= E.V u[5]= IDC.i Output Vector y: y[0]= T1.I y[1]= D1.I y[2]= T3.I y[3]= D3.I y[4]= Vo.V y[5]= L1.I y[6]= C1.V y[7]= E.I Parameter Vector p: p[0]= L1.L p[1]= L1.iL0 p[2]= C1.C p[3]= C1.vC0 p[4]= R1.r You can pause the simulation during running, change the Parameters you want and continue the Simulation
  FLYBACK_OS : Subsystem  mask{L1=1e-3, L2=4*1e-3, KP=1, C=1e-4, UC0=200, R=5}
      mask prompts: L1 "Inductance L1"; L2 "Inductance L2"; KP "Coupling Coeff"; C "Cap"; UC0 "initial Cap Voltage"; R "Load Resistance"
      mask help: Open Source Flyback Converter Input Vector u: u[0]= T1.gate u[1]= E.v u[2]= IDC.i Output Vector y: y[0]= T1.I y[1]= D1.I y[2]= Mut_L1.I y[3]= Mut_L1.V y[4]= Mut_L2.V y[5]= C1.V Parameter Vector p: p[0]= Mut_L1.L1 p[1]= Mut_L2.L2 p[2]= Mut_Coupling Coeff.k p[3]= C1.C p[4]= C1.vC0 p[5]= R1.r You can pause the simulation during running, change the Parameters you want and continue the Simulation
  FORWARD_OS : Subsystem  mask{L1=2e-3, L2=4*2e-3, L3=2e-3, KP1=1, KP2=1, KP3=1, L=1e-3, C=5e-4, UC0=100, R=5}
      mask prompts: L1 "Inductance L1"; L2 "Inductance L2"; L3 "Inductance L3"; KP1 "Coupling Coeff KP12"; KP2 "Coupling Coeff KP23"; KP3 "Coupling Coeff KP31"; L "Inductance"; C "Cap"; UC0 "initial Cap Voltage"; R "Load Resistance"
      mask help: Open Source forward Converter Input Vector u: u[0]= T1.gate u[1]= E.v u[2]= IDC.i Output Vector y: y[0]= T1.I y[1]= D1.I y[2]= L1.I y[3]= Mut_L1.V y[4]= Mut_L2.V y[5]= Mut_L3.V y[6]= D2.I y[7]= D3.I y[8]= C1.V Parameter Vector p: p[0]= Mut_L1.L1 p[1]= Mut_L2.L2 p[2]= Mut_L3.L3 p[3]= Mut_Coupling Coeff.k12 p[4]= Mut_Coupling Coeff.k23 p[5]= Mut_Coupling Coeff.k31 p[6]= L1.L p[7]= C1.C p[8]= C1.vC0 p[9]= R1.r You can pause the simulation during running, change the Parameters you want and continue the Simulation
  I2Q_OS : Subsystem  mask{L=5e-3, IL0=30, C=2e-4, VC0=50, R=10}
      mask prompts: L "Inductance L"; IL0 "Initial Ind. Current"; C "Capacitance"; VC0 "Initial Cap. Voltage"; R "Load Resistance"
      mask help: Current two Quadrant Converter Input Vector u: u[0]= T1.gate u[1]= T2.gate u[2]= E.v u[3]= IDC.i Output Vector y: y[0]= T1.I y[1]= T1.V y[2]= T2.I y[3]= T2.V y[4]= L1.I y[5]= C1.V y[6]= E.I Parameter Vector p: p[0]= L1.L p[1]= L1.iL0 p[2]= C1.C p[3]= C1.vC0 p[4]= R1.r You can pause the simulation during running, change the Parameters you want and continue the Simulation
  TS_FLYBACK_OS : Subsystem  mask{L1=1e-3, L2=4*1e-3, KP=1, C=5e-4, UC0=150, R=5}
      mask prompts: L1 "Inductance L1"; L2 "Inductance L2"; KP "Coupling Coeff KP"; C "Cap"; UC0 "initial Cap Voltage"; R "Load Resistance"
      mask help: Two Switchs Flyback Converter Input Vector u: u[0]= T1.gate and T2.gate u[1]= E.v u[2]= IDC.i Output Vector y: y[0]= T1.I y[1]= D1.I y[2]= T2.I y[3]= D2.I y[4]= D3.I y[5]= C1.V y[6]= E.I Parameter Vector p: p[0]= Mut_L1.L1 p[1]= Mut_L2.L2 p[2]= Mut_Coupling Coeff.k p[3]= C1.C p[4]= C1.vC0 p[5]= R1.r You can pause the simulation during running, change the Parameters you want and continue the Simulation
  TS_FORWARD_OS : Subsystem  mask{L1=2e-3, L2=4*2e-3, KP=1, L=5e-3, iL0=20, C=2e-4, UC0=100, R=5}
      mask prompts: L1 "Inductance L1"; L2 "Inductance L2"; KP "Coupling Coeff KP"; L "Inductance"; iL0 "Initial Ind. Current"; C "Cap"; UC0 "initial Cap Voltage"; R "Load Resistance"
      mask help: Two Switchs Forward Converter Input Vector u: u[0]= T1.gate and T2.gate u[1]= E.v u[2]= IDC.i Output Vector y: y[0]= T1.I y[1]= D1.I y[2]= T2.I y[3]= D2.I y[4]= L1.I y[5]= C1.V y[6]= E.I Parameter Vector p: p[0]= Mut_L1.L1 p[1]= Mut_L2.L2 p[2]= Mut_Coupling Coeff.k p[3]= L1.L p[4]= L1.iL10 p[5]= C1.C p[6]= C1.vC0 p[7]= R1.r You can pause the simulation during running, change the Parameters you want and continue the Simulation
  V2Q_OS : Subsystem  mask{L=5e-3, IL0=30, C=1e-4, VC0=50, R=10}
      mask prompts: L "Inductance L"; IL0 "Initial Current"; C "Capacitance C"; VC0 "Initial Cap Voltage VC0"; R "Load Resistance"
      mask help: Voltage two quadrant Converter Input Vector u: u[0]= T1.gate,T2.gate u[1]= E.v u[2]= IDC.i Output Vector y: y[0]= T1.I y[1]= D1.I y[2]= T2.I y[3]= D2.I y[4]= Vo.V y[5]= L1.I y[6]= C1.V y[7]= E.I Parameter Vector p: p[0]= L1.L p[1]= L1.iL0 p[2]= C1.C p[3]= C1.vC0 p[4]= R1.r You can pause the simulation during running, change the Parameters you want and continue the Simulation

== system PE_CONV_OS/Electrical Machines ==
  Asyn_M_model : Subsystem  mask{RR=0.228, LLR=0.8e-3, LM=34.7e-3, P=2}
      mask prompts: RR "Rotor Res."; LLR "Rotor Leakage Ind. (Refered)"; LM "Mag. Ind."; P "Pole Pairs"
      mask help: Machine-Model using the 3-phase stator currents and the mechanical angular velocity
  DCM_C_SF : Subsystem  mask(DCM C-S-Function Block
){Ra=.5, La=3e-3, Rf=200, Lf=1, If0=1, Laf=0.7, J=.0167, D=0.01, W0=0}
      mask prompts: Ra "Armature Resistance"; La "Armature Inductance"; Rf "Field Resistance"; Lf "Filed Inductance"; If0 "Initial field current"; Laf "Mutual Inductance"; J "Moment of Inertia"; D "Damping Coefficient"; W0 "initial ang. speed"
      mask help: Open source D-Motor modeled as Simulink C-S-Function Block Input Vector u: u[0]= Armature Voltage u[1]= Load Torque u[2]= Field Voltage Output Vector y: y[0]= Armature Current y[1]= EMF y[2]= Te y[3]= Ang. Velocity W Parameter Vector p: p[0]= Armature Resistance Ra p[1]= Armature Inductance La p[2]= Field Resistance Rf p[3]= Filed Inductance Lf p[4]= Initial field current ILf0 p[5]= Mutual Ind. Laf p[6]= Moment of Inertia J p[7]= Damp. Coef. D p[8]= Initial Ang. Velocity W0 You can pause the simulation during running, change the Parameters you want and continue the Simulation
  DCM_SL : Subsystem  mask(dcm){Ra=.5, La=3e-3, Rf=200, Lf=1, If0=1, Laf=0.7, J=.0167, D=0.01, omm0=0}
      mask prompts: Ra "Armature Resistance"; La "Armature Inductance"; Rf "Filed Resistance"; Lf "Filed Inductance"; If0 "Initial field current"; Laf "Mutual Inductance"; J "Moment of Inertia"; D "Damping Coefficient"; omm0 "initial ang. speed"
      mask help: Open source D-Motor modeled in Simulink Blocks Input Vector u: u[0]= Armature Voltage u[1]= Load Torque u[2]= Field Voltage Output Vector y: y[0]= Armature Current y[1]= EMF y[2]= Te y[3]= Ang. Velocity W Parameter Vector p: p[0]= Armature Resistance Ra p[1]= Armature Inductance La p[2]= Field Resistance Rf p[3]= Filed Inductance Lf p[4]= Initial field current ILf0 p[5]= Mutual Ind. Laf p[6]= Moment of Inertia J p[7]= Damp. Coef. D p[8]= Initial Ang. Velocity W0 You can pause the simulation during running, change the Parameters you want and continue the Simulation
  PM_SYNM_C_SF : Subsystem  mask(PSM-C-S-Function Block){R1=2.875, Lq=8.5e-3, Ld=8.5e-3, P=8, J=0.8e-3, D=0.5e-3, W0=0}
      mask prompts: R1 "Stator Resistance"; Lq "Q-Axis Inductance"; Ld "D-Axis Inductance"; P "Number of Poles"; J "Moment of Inertia"; D "Damping Coefficient"; W0 "initial ang. speed"
      mask help: Open source Permanent Magnet SYNCHRON MOTOR modeled as Simulink C-S-Function Blocks Input Vector u: u[0,1,2]= Three phase stator Voltages u[3]= Load Torque u[4]= PSI Output Vector y: y[0,1,2]= Three phase stator Currents y[3]= Te y[4]= Ang. Velocity W Parameter Vector p: p[0]= R1 p[1]= Lq p[2]= Ld p[3]= Number of Poles P p[4]= Moment of Inertia J p[5]= Damp. Coef. D p[6]= Initial Ang. Velocity W0 You can pause the simulation during running, change the Parameters you want and continue the Simulation
  PM_SYNM_SL : Subsystem  mask(PSM-SL){R1=2.875, Lq=8.5e-3, Ld=8.5e-3, P=8, J=0.8e-3, D=0.5e-3, omm0=0}
      mask prompts: R1 "Stator Resistance"; Lq "Q-Axis Inductance"; Ld "D-Axis Inductance"; P "Number of Poles"; J "Moment of Inertia"; D "Damping Coefficient"; omm0 "initial ang. speed"
      mask help: Open source Permanent Magnet SYNCHRON MOTOR modeled in Simulink Blocks Input Vector u: u[0,1,2]= Three phase stator Voltages u[3]= Load Torque u[4]= PSI Output Vector y: y[0,1,2]= Three phase stator Currents y[3]= Te y[4]= Ang. Velocity W Parameter Vector p: p[0]= R1 p[1]= Lq p[2]= Ld p[3]= Number of Poles P p[4]= Moment of Inertia J p[5]= Damp. Coef. D p[6]= Initial Ang. Velocity W0 You can pause the simulation during running, change the Parameters you want and continue the Simulation
  SC_ASYNM_SL : Subsystem  mask(SC_ASYN_MOTOR){rs=0.087, Lls=0.8e-3, rr=0.228, Llr=0.8e-3, Lm=34.7e-3, P=4, J=0.8, D=0.1, omm0=0}
      mask prompts: rs "Stator Resistance"; Lls "Stator Leakage Inductance"; rr "Rotor Resistance"; Llr "Rotor Leakage Inductance"; Lm "Magnetising Inductance"; P "Number of Poles"; J "Moment of Inertia"; D "Damping Coefficient"; omm0 "initial ang. speed"
      mask help: Open source Squirrel cage Asyn. MOTOR modeled in Simulink Blocks Input Vector u: u[0,1,2]= Three phase stator Voltages u[3]= Load Torque Output Vector y: y[0,1,2]= Three phase stator Currents y[3]= Te y[4]= Ang. Velocity W Parameter Vector p: p[0]= Rs p[1]= Ls p[2]= Rr p[3]= Lr p[4]= LM p[5]= Number of Poles P p[6]= Moment of Inertia J p[7]= Damp. Coef. D p[8]= Initial Ang. Velocity W0 You can pause the simulation during running, change the Parameters you want and continue the Simulation
  SC_AsynM_C_SF : Subsystem  mask(SC_ASYN_MOTOR){RS=0.087, LS=0.8e-3, RR=0.228, LR=0.8e-3, LM=34.7e-3, P=4, J=0.8, D=0.1, W0=0}
      mask prompts: RS "Stator Resistance"; LS "Stator Leakage Inductance"; RR "Rotor Resistance"; LR "Rotor Leakage Inductance"; LM "Magnetising Inductance"; P "Number of Poles"; J "Moment of Inertia"; D "Damping Coefficient"; W0 "initial ang. speed"
      mask help: Open source Squirrel cage Asyn. MOTOR modeled as Simulink C-S-Function Block Input Vector u: u[0,1,2]= Three phase stator Voltages u[3]= Load Torque Output Vector y: y[0,1,2]= Three phase stator Currents y[3]= Te y[4]= Ang. Velocity W Parameter Vector p: p[0]= Rs p[1]= Ls p[2]= Rr p[3]= Lr p[4]= LM p[5]= Number of Poles P p[6]= Moment of Inertia J p[7]= Damp. Coef. D p[8]= Initial Ang. Velocity W0 You can pause the simulation during running, change the Parameters you want and continue the Simulation
  SR_ASYNM_SL : Subsystem  mask(SR_Asyn_Motor_SL){rs=0.087, Lls=0.8e-3, rr=0.228, Llr=0.8e-3, Lm=34.7e-3, N12=1, P=4, J=0.8, D=0.1, omm0=0}
      mask prompts: rs "Stator Resistance"; Lls "Stator Leakage Inductance"; rr "Rotor Resistance'"; Llr "Rotor Leakage Inductance'"; Lm "Magnetising Inductance"; N12 "Turns Ratio"; P "Number of Poles"; J "Moment of Inertia"; D "Damping Coefficient"; omm0 "initial ang. speed"
      mask help: Open source Slip Ring Asyn. MOTOR modeled in Simulink Blocks Input Vector u: u[0,1,2]= Three phase stator Voltages u[3,4,5]= Three phase Rotor Voltages u[6]= Load Torque Output Vector y: y[0,1,2]= Three phase stator Currents y[3,4,5]= Three phase Rotor Currents y[6]= Te y[7]= Ang. Velocity W Parameter Vector p: p[0]= Rs p[1]= Ls p[2]= Rr p[3]= Lr p[4]= LM p[5]= Turns Ratio p[6]= Number of Poles P p[7]= Moment of Inertia J p[8]= Damp. Coef. D p[9]= Initial Ang. Velocity W0 You can pause the simulation during running, change the Parameters you want and continue the Simulation
  SR_AsynM_C_SF : Subsystem  mask(SR_ASYN_MOTOR_C-SF){RS=0.087, LS=0.8e-3, RR=0.228, LR=0.8e-3, LM=34.7e-3, N12=1, P=4, J=0.8, D=0.1, W0=0}
      mask prompts: RS "Stator Resistance"; LS "Stator Leakage Inductance"; RR "Rotor Resistance"; LR "Rotor Leakage Inductance"; LM "Magnetising Inductance"; N12 "Turns ratio"; P "Number of Poles"; J "Moment of Inertia"; D "Damping Coefficient"; W0 "initial ang. speed"
      mask help: Open source Slip Ring Asyn. MOTOR modeled as Simulink C-S-Function Block Input Vector u: u[0,1,2]= Three phase stator Voltages u[3,4,5]= Three phase Rotor Voltages u[6]= Load Torque Output Vector y: y[0,1,2]= Three phase stator Currents y[3,4,5]= Three phase Rotor Currents y[6]= Te y[7]= Ang. Velocity W Parameter Vector p: p[0]= Rs p[1]= Ls p[2]= Rr p[3]= Lr p[4]= LM p[5]= Turns Ratio p[6]= Number of Poles P p[7]= Moment of Inertia J p[8]= Damp. Coef. D p[9]= Initial Ang. Velocity W0 You can pause the simulation during running, change the Parameters you want and continue the Simulation
  SYNM_C_SF : Subsystem  mask(Syn. MOTOR C-S-Function Block){rs=0.1, Lls=0.79e-3, rk=0.17, Llkq=0.91e-3, Llkd=0.29e-3, Lmq=2e-3, Lmd=4.1e-3, rf=.16, Llf=0.38e-3, P=4, J=.2, D=0.05}
      mask prompts: rs "Stator Resistance"; Lls "Stator Leakage Inductance"; rk "Damper Winding Resistance"; Llkq "Damper Q-Axis Leakage Inductance"; Llkd "Damper D-Axis Leakage Inductance"; Lmq "Q-Axis Magnetising Inductance"; Lmd "D-Axis Magnetising Inductance"; rf "Field  Winding Resistance"; Llf "Field Winding Leakage Inductance"; P "Number of Poles"; J "Moment of Inertia"; D "Damping Coefficient"
      mask help: Open source Syn. MOTOR modeled as Simulink C-S-Function Block Input Vector u: u[0,1,2]= Three phase stator Voltages u[3] = Field DC-Voltages u[4] = Load Torque Output Vector y: y[0,1,2]= Three phase stator Currents y[3]= Te y[4]= Ang. Velocity W y[5]= Field DC-Current Parameter Vector p: p[0]= Stator Resistance rs p[1]= Stator Leakage Inductance Lls p[2]= Damper Winding Resistance rk p[3]= Damper Q-Axis Leakage Inductance Llkq p[4]= Damper D-Axis Leakage Inductance Llkd p[5]= Q-Axis Magnetising Inductance Lmq p[6]= D-Axis Magnetising Inductance Lmd p[7]= Field Winding Resistance rf p[8]= Field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
  SYNM_SL : Subsystem  mask(Syn. MOTOR Simulink Blocks){rs=0.1, Lls=0.79e-3, rk=0.17, Llkq=0.91e-3, Llkd=0.29e-3, Lmq=2e-3, Lmd=4.1e-3, rf=.16, Llf=0.38e-3, P=4, J=.2, D=0.05, omm0=0}
      mask prompts: rs "Stator Resistance"; Lls "Stator  Leakage Inductance"; rk "Damper Winding Resistance"; Llkq "Damper Q-Axis Leakage Inductance"; Llkd "Damper D-Axis Leakage Inductance"; Lmq "Q-Axis Magnetising Inductance"; Lmd "D-Axis Magnetising Inductance"; rf "Field  Winding Resistance"; Llf "Field Winding Leakage Inductance"; P "Number of Poles"; J "Moment of Inertia"; D "Damping Coefficient"; omm0 "initial ang. speed"
      mask help: Open source Syn. MOTOR modeled in Simulink Blocks Input Vector u: u[0,1,2]= Three phase stator Voltages u[3] = Field DC-Voltages u[4] = Load Torque Output Vector y: y[0,1,2]= Three phase stator Currents y[3]= Te y[4]= Ang. Velocity W y[5]= Field DC-Current Parameter Vector p: p[0]= Stator Resistance rs p[1]= Stator Leakage Inductance Lls p[2]= Damper Winding Resistance rk p[3]= Damper Q-Axis Leakage Inductance Llkq p[4]= Damper D-Axis Leakage Inductance Llkd p[5]= Q-Axis Magnetising Inductance Lmq p[6]= D-Axis Magnetising Inductance Lmd p[7]= Field Winding Resistance rf p[8]= Field Winding Lea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
  abc/dq0k : Subsystem
  abc/dq0s : Subsystem
  abc/p(t) : Subsystem
  abc/q(t) : Subsystem
  abc/qd0k : Subsystem
  abc/qd0s : Subsystem
  dq0k/abc : Subsystem
  dq0s/abc : Subsystem
  dqk/dqs : Subsystem
  dqs/dqk : Subsystem
  qd0k/abc : Subsystem
  qd0s/abc : Subsystem
  qdk/qds : Subsystem
  qds/qdk : Subsystem
  th : Subsystem

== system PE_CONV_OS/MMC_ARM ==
  MMC-CDSM_ARM : Subsystem  mask(MMC_CDSM_ARM){C=C, UC0=UC0, Nc=Nc}
      mask prompts: C "C [F]"; UC0 "UC0 [V]"; Nc "Number Caps"
      mask help: Input Vector Switching Signals Arm Current Output Vector Capacitor Voltages Capacitor Current IT1, ID1, VT1, IT2, ID2, VT2 Arm Voltage Parameter Vector Capacitor Value =p[0] Initial Capacitor Voltage =p[1] Number of Cap. =p[2]
  MMC-FB_ARM : Subsystem  mask(MMC_FB_ARM){C=C, UC0=UC0, Nc=Nc}
      mask prompts: C "C [F]"; UC0 "UC0 [V]"; Nc "Number Caps"
      mask help: Input Vector Switching Signals Arm Current Output Vector Capacitor Voltages Capacitor Current IT1, ID1, VT1, IT2, ID2, VT2 Arm Voltage Parameter Vector Capacitor Value =p[0] Initial Capacitor Voltage =p[1] Number of Cap. =p[2]
  MMC-HB_ARM : Subsystem  mask(MMC_HB_ARM){C=C, UC0=UC0, Nc=Nc}
      mask prompts: C "C [F]"; UC0 "UC0 [V]"; Nc "Number Caps"
      mask help: Input Vector Switching Signals Arm Current Output Vector Capacitor Voltages Capacitor Current IT1, ID1, VT1, IT2, ID2, VT2 Arm Voltage Parameter Vector Capacitor Value =p[0] Initial Capacitor Voltage =p[1] Number of Cap. =p[2]
